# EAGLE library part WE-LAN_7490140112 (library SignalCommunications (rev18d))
WE-LAN LAN Transformer 10/100 Base T - Compliant with IEEE 802.3, IEEE 802.3af and IEEE 802.3at standards - SMT -- Ethernet -- Power over Ethernet -- 1 Gigabit Ethernet -- Compliant with most IC's for ethernet applications like Intel, AMD, Globespan and Realtek -- Hub, Router, Switch Details see: http://katalog.we-online.de/en/pbs/WE-LAN/7490140112 2016 (C) Würth Elektronik
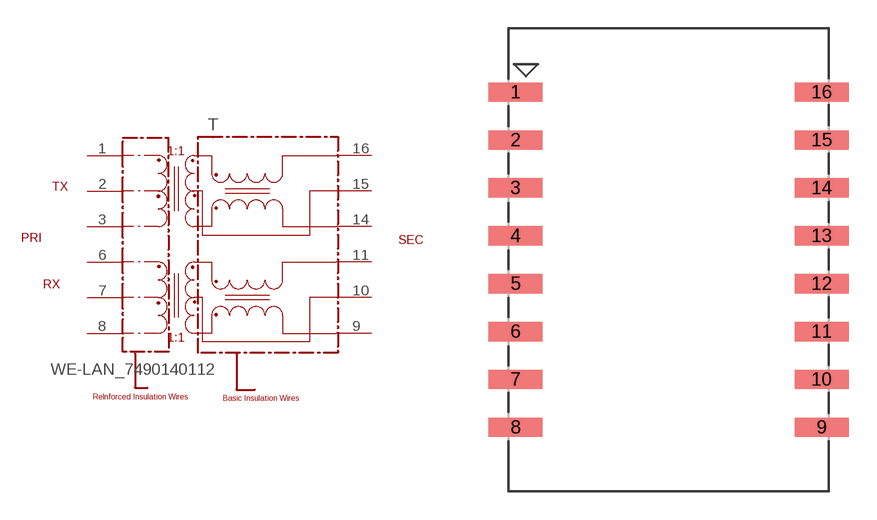
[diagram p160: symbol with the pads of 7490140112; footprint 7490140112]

Designator prefix T

## WE-LAN_7490140112  [7490140112]
1  1
2  2
3  3
6  6
7  7
8  8
9  9
10  10
11  11
14  14
15  15
16  16

## Footprint 7490140112 (pad centres in mm)
smd 2.87 x 1.02: 1 -8.115,8.89; 2 -8.115,6.35; 3 -8.115,3.81; 4 -8.115,1.27; 5 -8.115,-1.27; 6 -8.115,-3.81; 7 -8.115,-6.35; 8 -8.115,-8.89; 9 8.115,-8.89; 10 8.115,-6.35; 11 8.115,-3.81; 12 8.115,-1.27; 13 8.115,1.27; 14 8.115,3.81; 15 8.115,6.35; 16 8.115,8.89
